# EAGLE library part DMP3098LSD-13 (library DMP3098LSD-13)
MOSFET PMOS-DUAL Source: Datasheet
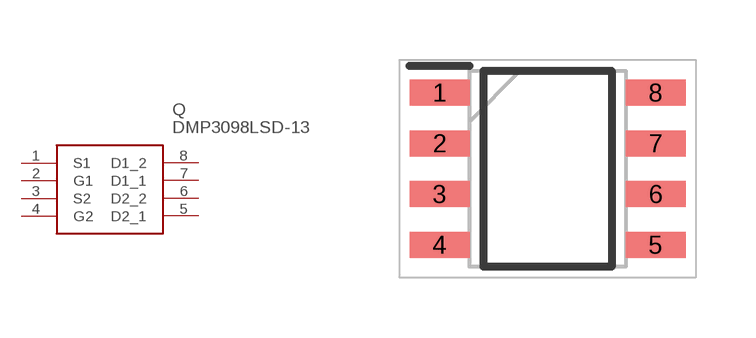
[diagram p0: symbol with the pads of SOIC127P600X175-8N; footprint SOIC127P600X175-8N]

Designator prefix Q

## DMP3098LSD-13 (Description: MOSFET PMOS-DUAL; Height: 1.75mm; Manufacturer_Name: Diodes Incorporated; Manufacturer_Part_Number: DMP3098LSD-13; Mouser_Part_Number: 621-DMP3098LSD-13; Mouser_Price-Stock: https://www.mouser.co.uk/ProductDetail/Diodes-Incorporated/DMP3098LSD-13?qs=oUsD4qhOtFxafARAi3NzqQ%3D%3D)  [SOIC127P600X175-8N]
1  S1
2  G1
3  S2
4  G2
5  D2_1
6  D2_2
7  D1_1
8  D1_2

## Footprint SOIC127P600X175-8N (pad centres in mm)
SO-8
smd 1.5 x 0.65: 1 -2.7,1.905; 2 -2.7,0.635; 3 -2.7,-0.635; 4 -2.7,-1.905; 5 2.7,-1.905; 6 2.7,-0.635; 7 2.7,0.635; 8 2.7,1.905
